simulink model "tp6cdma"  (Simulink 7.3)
settings: Solver=ode45  StartTime=0.0  StopTime=10.0  RelTol=1e-3
undefined symbols (not defined in the file or in its folder): array, Concatenate, D, fe1, fe2, frames
libraries: commdigbbndpm3 x4, commutil2 x2, dspbuff3 x2, commseqgen2 x2, commfilt2 x2, dspsrcs4 x2, dspsnks4 x2, commchan3 x1

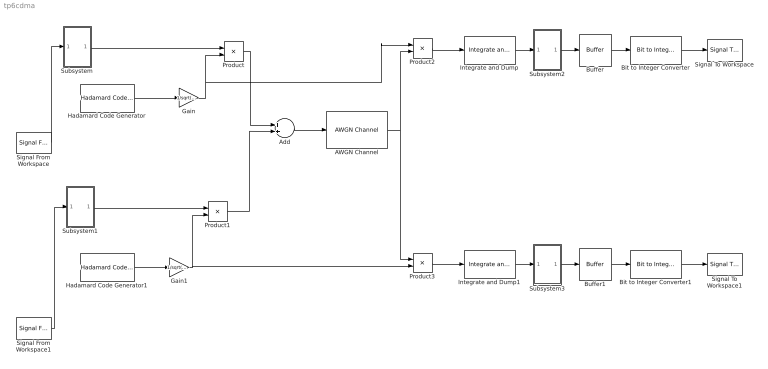
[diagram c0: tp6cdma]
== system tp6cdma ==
  AWGN Channel : commchan3/AWGN Channel  SystemSampleTime=-1  seed=1237  noiseMode="Signal to noise ratio  (SNR)"  EbNodB=10  EsNodB=10  SNRdB=20  bitsPerSym=1  Ps=1  Tsym=1  variance=1
  Add : Sum  OutDataType=fixdt(1, 16)  OutScaling=2^-10
  Bit to Integer Converter : commutil2/Bit to Integer Converter  nbits=8  bitOrder=MSB first  signedOutputValues=Unsigned  outDtype=uint8  outDtypeSigned=Inherit via internal rule
  Bit to Integer Converter1 : commutil2/Bit to Integer Converter  nbits=8  bitOrder=MSB first  signedOutputValues=Unsigned  outDtype=uint8  outDtypeSigned=Inherit via internal rule
  Buffer : dspbuff3/Buffer  N=8  V=0  ic=0
  Buffer1 : dspbuff3/Buffer  N=8  V=0  ic=0
  Gain : Gain  Gain=1/sqrt(64)  ParameterDataType=fixdt(1, 16)  ParameterScaling=2^0  OutDataType=fixdt(1, 16)  OutScaling=2^0
  Gain1 : Gain  Gain=1/sqrt(64)  ParameterDataType=fixdt(1, 16)  ParameterScaling=2^0  OutDataType=fixdt(1, 16)  OutScaling=2^0
  Hadamard Code Generator : commseqgen2/Hadamard Code Generator  SystemSampleTime=-1  length=64  index=30  ts=1/(64*fe1)  frameBased=on  sampPerFrame=64  outDataType=double
  Hadamard Code Generator1 : commseqgen2/Hadamard Code Generator  SystemSampleTime=-1  length=64  index=11  ts=1/(64*fe2)  frameBased=on  sampPerFrame=64  outDataType=double
  Integrate and Dump : commfilt2/Integrate and Dump  DialogController=commDDGCreate  DialogControllerArgs=DataTag0  obssamples=64  offsetsamples=0  nodump=off  roundingMode=Floor  overflowMode=off
  Integrate and Dump1 : commfilt2/Integrate and Dump  DialogController=commDDGCreate  DialogControllerArgs=DataTag1  obssamples=64  offsetsamples=0  nodump=off  roundingMode=Floor  overflowMode=off
  Product{,1..3} (4 alike) : Product  OutDataType=fixdt(1, 16)  OutScaling=2^0
  Signal From Workspace : dspsrcs4/Signal From Workspace  SystemSampleTime=-1  X=fy  Ts=1/(8*fe1)  nsamps=1  OutputAfterFinalValue=Cyclic repetition  ignoreOrWarnInputAndFrameLengths=on
  Signal From Workspace1 : dspsrcs4/Signal From Workspace  SystemSampleTime=-1  X=fx  Ts=1/(8*fe2)  nsamps=1  OutputAfterFinalValue=Cyclic repetition  ignoreOrWarnInputAndFrameLengths=on
  Signal To Workspace : dspsnks4/Signal To Workspace  SystemSampleTime=-1  VariableName=yout1  FrameMode=Concatenate frames (2-D array)
  Signal To Workspace1 : dspsnks4/Signal To Workspace  SystemSampleTime=-1  VariableName=yout2  FrameMode=Concatenate frames (2-D array)
  Subsystem : Subsystem
  Subsystem1 : Subsystem
  Subsystem2 : Subsystem
  Subsystem3 : Subsystem
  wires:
  Signal From Workspace/1 -> Subsystem/1(In1)
  Signal From Workspace1/1 -> Subsystem1/1(In1)
  Hadamard Code Generator/1 -> Gain/1
  Gain/1 -> Product/2, Product2/1
  Subsystem/1(Out1) -> Product/1
  Hadamard Code Generator1/1 -> Gain1/1
  Gain1/1 -> Product1/2, Product3/2
  Subsystem1/1(Out1) -> Product1/1
  Product/1 -> Add/1
  Product1/1 -> Add/2
  Add/1 -> AWGN Channel/1
  AWGN Channel/1 -> Product3/1, Product2/2
  Product2/1 -> Integrate and Dump/1
  Product3/1 -> Integrate and Dump1/1
  Integrate and Dump/1 -> Subsystem2/1(In1)
  Subsystem2/1(Out1) -> Buffer/1
  Integrate and Dump1/1 -> Subsystem3/1(In1)
  Subsystem3/1(Out1) -> Buffer1/1
  Buffer1/1 -> Bit to Integer Converter1/1
  Buffer/1 -> Bit to Integer Converter/1
  Bit to Integer Converter1/1 -> Signal To Workspace1/1
  Bit to Integer Converter/1 -> Signal To Workspace/1

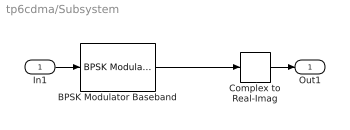
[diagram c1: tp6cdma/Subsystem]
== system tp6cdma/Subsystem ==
  In1 : Inport
  BPSK Modulator Baseband : commdigbbndpm3/BPSK Modulator Baseband  DialogController=commDDGCreate  DialogControllerArgs=DataTag2  SystemSampleTime=-1  Ph=0  outDtype=double  outWordLen=16  outUDDataType=sfix(16)  outFracLenMode=Best precision  outFracLen=15
  Complex to Real-Imag : ComplexToRealImag  Output=Real
  Out1 : Outport
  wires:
  BPSK Modulator Baseband/1 -> Complex to Real-Imag/1
  In1/1 -> BPSK Modulator Baseband/1
  Complex to Real-Imag/1 -> Out1/1

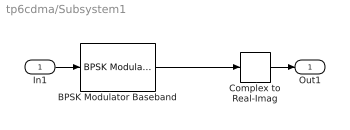
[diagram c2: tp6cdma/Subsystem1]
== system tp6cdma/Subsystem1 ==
  In1 : Inport
  BPSK Modulator Baseband : commdigbbndpm3/BPSK Modulator Baseband  DialogController=commDDGCreate  DialogControllerArgs=DataTag3  SystemSampleTime=-1  Ph=0  outDtype=double  outWordLen=16  outUDDataType=sfix(16)  outFracLenMode=Best precision  outFracLen=15
  Complex to Real-Imag : ComplexToRealImag  Output=Real
  Out1 : Outport
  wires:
  BPSK Modulator Baseband/1 -> Complex to Real-Imag/1
  In1/1 -> BPSK Modulator Baseband/1
  Complex to Real-Imag/1 -> Out1/1

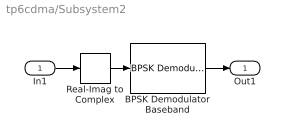
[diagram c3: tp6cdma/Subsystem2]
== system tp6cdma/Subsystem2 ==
  In1 : Inport
  BPSK Demodulator Baseband : commdigbbndpm3/BPSK Demodulator Baseband  DialogController=commDDGCreate  DialogControllerArgs=DataTag4  Ph=0  DecType=Hard decision  VarSource=Dialog  Variance=1  outDtype=Inherit via internal rule  derotateFactorWordLen=16
  Real-Imag to Complex : RealImagToComplex  Input=Real
  Out1 : Outport
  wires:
  Real-Imag to Complex/1 -> BPSK Demodulator Baseband/1
  BPSK Demodulator Baseband/1 -> Out1/1
  In1/1 -> Real-Imag to Complex/1

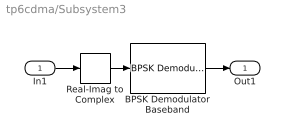
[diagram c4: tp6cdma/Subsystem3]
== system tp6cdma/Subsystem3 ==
  In1 : Inport
  BPSK Demodulator Baseband : commdigbbndpm3/BPSK Demodulator Baseband  DialogController=commDDGCreate  DialogControllerArgs=DataTag5  Ph=0  DecType=Hard decision  VarSource=Dialog  Variance=1  outDtype=Inherit via internal rule  derotateFactorWordLen=16
  Real-Imag to Complex : RealImagToComplex  Input=Real
  Out1 : Outport
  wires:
  Real-Imag to Complex/1 -> BPSK Demodulator Baseband/1
  BPSK Demodulator Baseband/1 -> Out1/1
  In1/1 -> Real-Imag to Complex/1
